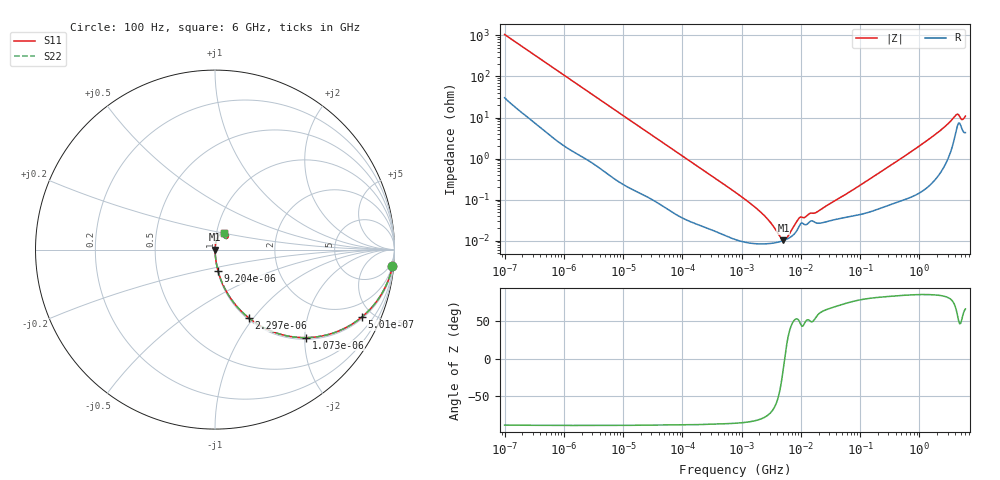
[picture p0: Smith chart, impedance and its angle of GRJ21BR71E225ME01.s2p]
!Murata Part Number: GRJ21BR71E225ME01
!These Parameters are Measured in Series Mode Connection
!Data Generated on Jun 19, 2026
!  o--ll--o
!Port1  Port2
!  o------o
!Operation Temp=25[degC], DC Bias Voltage=0[V]
!Freq. Start=100[Hz] Stop=6[GHz] 401[Steps]
# Hz S RI R 50
!Freq.(Hz) S11(Real) S11(Imag) S21(Real) S21(Imag) S12(Real) S12(Imag) S22(Real) S22(Imag)
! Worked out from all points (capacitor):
!   401 points, 100 Hz to 6 GHz, reference 50 ohm
!   read as one part in series: C = 1.5 uF near 109 Hz
!   lowest |Z| = 10.3 mohm at 5.079 MHz (marker M1)
!   series resonance near 5.326 MHz, so ESL is about 600 pH
!   S11 on the Smith chart (normalised r, x): 100 Hz: 2, -21; 501 Hz: 1.09, -4.30; 1.073 kHz: 1.04, -2.02; 2.297 kHz: 1.02, -0.95; 9.204 kHz: 1.01, -0.24; 6 GHz: 1.09, +0.20
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100  0.9885 -0.0933  0.0115 0.0933  0.0115 0.0933  0.9885 -0.0933
268  0.9363 -0.233  0.0637 0.233  0.0637 0.233  0.9363 -0.233
501  0.8174 -0.3762  0.1826 0.3762  0.1826 0.3762  0.8174 -0.3762
1073  0.5061 -0.4906  0.4939 0.4906  0.4939 0.4906  0.5061 -0.4906
2008  0.2334 -0.4129  0.7666 0.4129  0.7666 0.4129  0.2334 -0.4129
2297  0.1905 -0.3824  0.8095 0.3824  0.8095 0.3824  0.1905 -0.3824
4111  0.072 -0.2481  0.928 0.2481  0.928 0.2481  0.072 -0.2481
9204  0.0169 -0.1189  0.9831 0.1189  0.9831 0.1189  0.0169 -0.1189
40335  0.00159 -0.0282  0.9984 0.0282  0.9984 0.0282  0.00159 -0.0282
774597  0.000109 -0.00152  0.9999 0.00152  0.9999 0.00152  0.000109 -0.00152
2372521  8.33e-05 -0.000411  0.9999 0.000411  0.9999 0.000411  8.33e-05 -0.000411
5079039  0.0001 -2.18e-05  0.9999 2.18e-05  0.9999 2.18e-05  0.0001 -2.18e-05
5809218  0.000108 4.03e-05  0.9999 -4.03e-05  0.9999 -4.03e-05  0.000108 4.03e-05
9506416  0.000233 0.000276  0.9998 -0.000276  0.9998 -0.000276  0.000233 0.000276
1.555665e7  0.000303 0.000355  0.9997 -0.000355  0.9997 -0.000355  0.000303 0.000355
1.946e7  0.000265 0.000442  0.9997 -0.000442  0.9997 -0.000442  0.000265 0.000442
3.124326e8  0.000779 0.00645  0.9992 -0.00645  0.9992 -0.00645  0.000779 0.00645
1.791126e9  0.00423 0.0367  0.9958 -0.0367  0.9958 -0.0367  0.00423 0.0367
4.009986e9  0.0438 0.0947  0.9562 -0.0947  0.9562 -0.0947  0.0438 0.0947
4.385646e9  0.067 0.091  0.933 -0.091  0.933 -0.091  0.067 0.091
5.245841e9  0.0546 0.064  0.9454 -0.064  0.9454 -0.064  0.0546 0.064
6e9  0.0497 0.0905  0.9503 -0.0905  0.9503 -0.0905  0.0497 0.0905
